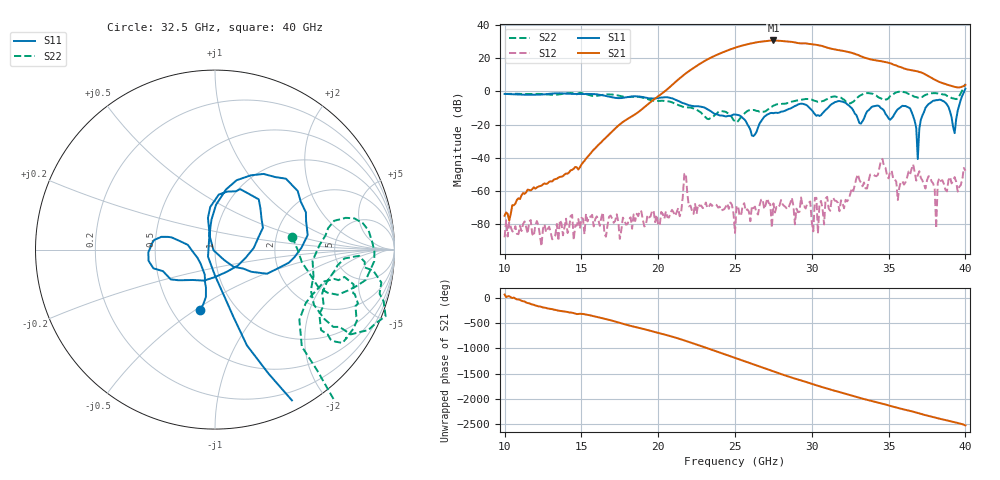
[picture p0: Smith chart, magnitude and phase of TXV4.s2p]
!Keysight Technologies,M9808A,MY58100618,A.14.70.03
!Date: Monday, February 27, 2023 13:19:05
!Correction: S11(C  2-Port  )
!S21(C  2-Port  )
!S12(C  2-Port  )
!S22(C  2-Port  )
!S2P File: Measurements: S11, S21, S12, S22:
# Hz S  RI  R 50
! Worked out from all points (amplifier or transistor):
!   301 points, 10 GHz to 40 GHz, reference 50 ohm
!   highest |S21| = 30.7 dB at 27.5 GHz (marker M1)
!   |S21| within 3 dB of that: 25.5 GHz to 30.53 GHz (5.035 GHz wide, 18 % of centre)
!   unconditionally stable (mu >= 1): start of sweep to 35.72 GHz; 35.89 GHz to 39.77 GHz
!   at 15 GHz: K = 29476.40, MAG = -31.7 dB, |S12| = -76.1 dB
!   at 25 GHz: K = 411.73, MAG = 26.5 dB, |S12| = -85.1 dB
!   at 40 GHz: K = 64.67, MSG = 25.8 dB, |S12| = -47.7 dB
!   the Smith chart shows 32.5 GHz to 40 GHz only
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1e10  0.7224 0.4318  8.42e-05 0.000162  1.68e-05 -3.74e-05  0.129 0.8253
1.5e10  0.6359 -0.5421  0.00471 0.00417  0.000148 5.19e-05  0.6744 0.5939
2e10  -0.2187 -0.5952  0.6463 0.3029  -9.16e-05 -2.07e-05  0.1959 -0.4788
2.25e10  -0.3452 -0.1006  -5.329 2.38  0.000159 0.000134  -0.0318 -0.2805
2.34e10  -0.2501 -0.0631  4.896 9.009  -0.000391 -0.000145  -0.1103 -0.1133
2.42e10  -0.1783 0.0578  13.78 -5.864  5.81e-05 -0.000269  -0.2095 -0.1431
2.5e10  -0.1399 0.1468  -6.175 -19.69  1.39e-05 -5.37e-05  -0.1217 -0.0411
2.58e10  -0.0579 0.086  -25.37 6.018  0.000206 -0.000196  -0.2021 0.1564
2.65e10  0.0823 -0.00526  -1.313 30.52  0.000198 1.28e-05  -0.1907 0.174
2.69e10  0.1615 -0.0628  20.93 24.64  0.000281 -6.21e-05  -0.0975 0.2256
2.75e10  0.1838 -0.1233  32.98 -8.79  -5.78e-05 -0.000425  -0.000705 0.3721
2.82e10  0.1135 -0.2308  1.116 -32.51  -0.000211 0.000292  0.0653 0.4203
2.89e10  0.0346 -0.3617  -27.35 -11.49  -4.94e-06 -0.000101  0.2308 0.4639
2.95e10  0.0781 -0.4042  -24.01 14.5  0.000217 0.000276  0.2002 0.5438
3e10  0.0611 -0.2661  -4.356 25.94  -6.15e-05 9.5e-05  0.1785 0.5367
3.08e10  -0.199 -0.1459  20.6 8.389  -6.83e-05 -7.26e-05  0.4329 0.3006
3.19e10  -0.2676 -0.4245  5.502 -16.1  -0.000267 -0.000463  0.5097 0.3985
3.3e10  -0.0571 -0.1392  -12.33 -2.421  0.00158 -0.0028  0.6268 -0.2406
3.4e10  -0.3546 0.0299  -3.767 7.994  -0.001 0.00296  0.8241 0.1467
3.5e10  -0.000804 -0.1535  6.006 4.008  -0.000143 0.00242  0.5514 -0.3082
3.64e10  0.0211 0.3068  1.096 -4.295  -0.00221 0.00235  0.8347 -0.069
4e10  0.5479 -1.083  1.577 -0.0548  0.00284 -0.003  1.032 -1.32
